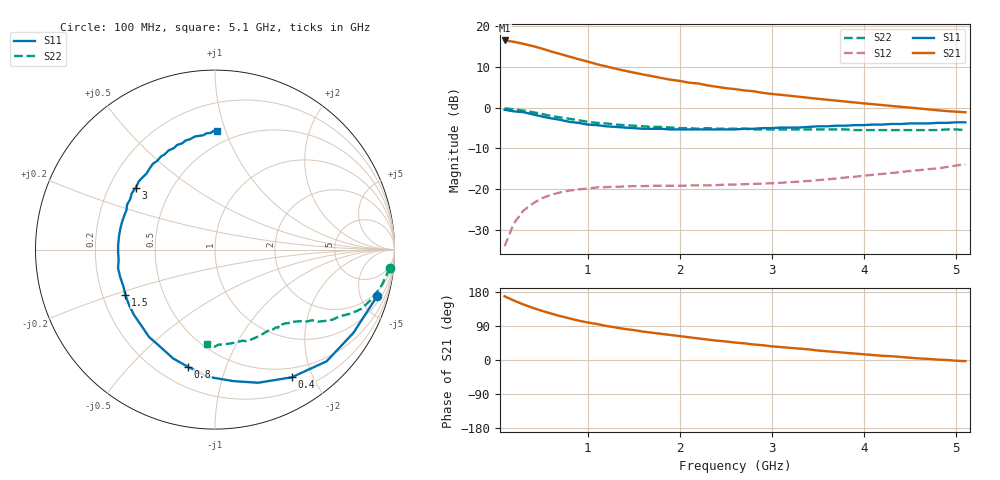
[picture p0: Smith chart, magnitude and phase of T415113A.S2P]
!AT-41511
!S and NOISE PARAMETERS at Vce=2.7V  Ic=2mA.  LAST UPDATED 01-25-95
# ghz s ma r 50
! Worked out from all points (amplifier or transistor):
!   51 points, 100 MHz to 5.1 GHz, reference 50 ohm
!   highest |S21| = 16.5 dB at 100 MHz (marker M1)
!   |S21| within 3 dB of that: start of sweep to 651.7 MHz
!   unconditionally stable (mu >= 1): 2.192 GHz to 4.94 GHz
!   at 900 MHz: K = 0.44, MSG = 16.0 dB, |S12| = -20.1 dB
!   at 2.6 GHz: K = 1.12, MAG = 9.6 dB, |S12| = -18.9 dB
!   at 5.1 GHz: K = 0.98, MSG = 6.4 dB, |S12| = -13.9 dB
!   lowest NFmin = 0.80 dB at 100 MHz
!   S11 on the Smith chart (normalised r, x): 100 MHz: 1.52, -6.78; 400 MHz: 0.37, -1.71; 800 MHz: 0.31, -0.75; 1.5 GHz: 0.30, -0.22; 3 GHz: 0.31, +0.31; 5.1 GHz: 0.40, +0.93
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0.1  0.94 -16.0  6.658 168.0  0.02 81.0  0.98 -6.0
0.2  0.9 -31.0  6.418 157.0  0.038 72.0  0.95 -12.0
0.3  0.88 -45.0  6.058 147.0  0.054 65.0  0.92 -17.0
0.4  0.83 -59.0  5.705 138.0  0.066 58.0  0.88 -22.0
0.5  0.78 -72.0  5.312 130.0  0.077 52.0  0.84 -25.0
0.6  0.74 -82.0  4.893 123.0  0.085 47.0  0.79 -28.0
0.7  0.71 -93.0  4.552 116.0  0.091 43.0  0.76 -31.0
0.8  0.67 -103.0  4.225 110.0  0.096 39.0  0.73 -33.0
0.9  0.65 -111.0  3.929 104.0  0.099 37.0  0.7 -35.0
1  0.62 -120.0  3.67 99.0  0.102 35.0  0.67 -36.0
1.2  0.59 -134.0  3.2 90.0  0.106 31.0  0.64 -39.0
1.4  0.57 -147.0  2.837 82.0  0.108 28.0  0.61 -41.0
1.5  0.56 -153.0  2.691 79.0  0.109 28.0  0.6 -42.0
1.6  0.55 -158.0  2.552 75.0  0.109 27.0  0.59 -43.0
1.8  0.55 -169.0  2.305 69.0  0.11 26.0  0.58 -45.0
2.2  0.54 172.0  1.975 57.0  0.111 27.0  0.55 -50.0
2.4  0.54 164.0  1.801 51.0  0.112 28.0  0.55 -52.0
2.6  0.54 156.0  1.686 46.0  0.114 28.0  0.55 -55.0
3  0.56 142.0  1.47 36.0  0.118 31.0  0.54 -60.0
3.5  0.59 126.0  1.283 25.0  0.129 36.0  0.54 -67.0
4.3  0.63 105.0  1.047 10.0  0.158 39.0  0.53 -79.0
5.1  0.66 89.0  0.877 -3.0  0.202 40.0  0.53 -95.0
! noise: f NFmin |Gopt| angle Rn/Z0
0.1  0.8  0.65  5  0.4
0.9  1  0.55  62  0.26
1.8  1.4  0.45  129  0.13
2.4  1.7  0.48  168  0.09
